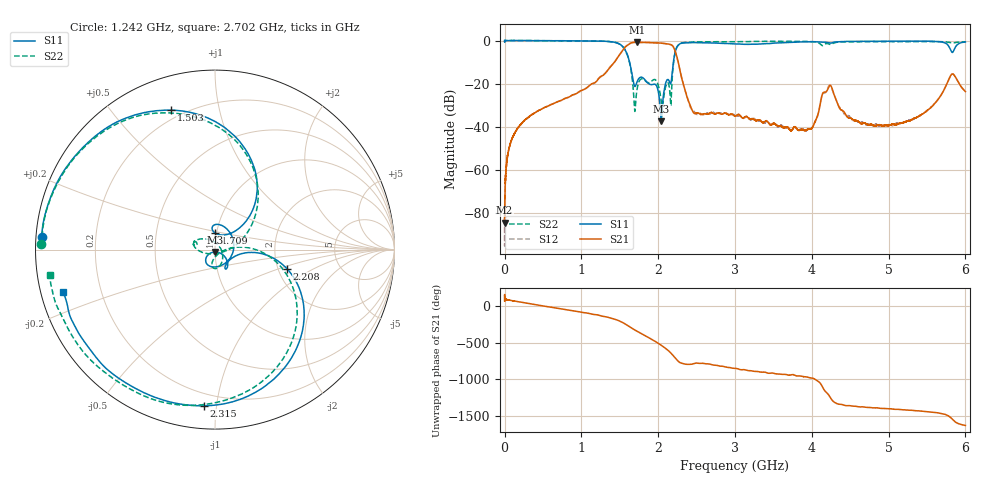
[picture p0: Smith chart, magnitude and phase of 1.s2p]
!Keysight Technologies,N5232A,MY52221221,A.10.65.11
!Date: Sunday, April 23, 2023 11:18:08
!Correction: S11(Full 2 Port(1,4))
!S41(Full 2 Port(1,4))
!S14(Full 2 Port(1,4))
!S44(Full 2 Port(1,4))
!S2P File: Measurements: S11, S41, S14, S44:
# Hz S  RI  R 50
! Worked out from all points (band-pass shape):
!   16001 points, 300 kHz to 6 GHz, reference 50 ohm
!   highest |S21| = -0.83 dB at 1.722 GHz (marker M1); lowest = -84.6 dB at 675 kHz (marker M2)
!   |S21| within 3 dB of the highest: 1.551 GHz to 2.209 GHz (658.2 MHz wide, 35 % of centre)
!   lowest |S11| = -37.5 dB at 2.039 GHz (marker M3), VSWR 1.03, Z = 50 - j1.33 ohm
!   |S11| at or under -10 dB: 1.627 GHz to 2.198 GHz (571.1 MHz wide, 29.9 % of centre)
!   |S22| runs from -32.9 to 0.0 dB; largest |S21 - S12| = 0.024
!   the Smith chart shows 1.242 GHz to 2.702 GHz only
!   S11 on the Smith chart (normalised r, x): 1.242 GHz: 0.02, +0.04; 1.503 GHz: 0.16, +0.72; 1.709 GHz: 0.99, +0.18; 2.208 GHz: 2.23, -0.57; 2.315 GHz: 0.13, -0.93; 2.702 GHz: 0.07, -0.14
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300000  0.999 -0.00352  2.45e-05 6.59e-05  8.74e-05 6.44e-05  0.9988 -0.00308
674981.2  0.9223 0.0318  -5.34e-05 2.5e-05  6.53e-07 -1.69e-05  0.9179 0.042
5.542224e7  0.9858 -0.1449  0.000553 0.00299  0.000502 0.00295  0.986 -0.141
1.780411e8  0.8867 -0.4586  0.00526 0.00818  0.00523 0.00813  0.894 -0.4466
1.000375e9  -0.816 -0.5428  0.00475 -0.0695  0.00649 -0.0679  -0.7934 -0.5667
1.241863e9  -0.9663 0.0703  -0.0925 -0.1079  -0.092 -0.1037  -0.9681 0.0285
1.50285e9  -0.2463 0.7769  -0.4234 0.2386  -0.4193 0.2331  -0.2972 0.762
1.708715e9  0.00118 0.0917  0.8254 0.3764  0.8298 0.3732  -0.0345 -0.0232
1.722214e9  -0.0127 0.106  0.8713 0.257  0.8734 0.251  -0.067 -0.0167
1.877456e9  0.0972 -0.0225  0.2656 -0.8616  0.2678 -0.8536  -0.102 0.0259
2.00045e9  -0.0491 -0.045  -0.75 -0.4556  -0.7498 -0.4571  -0.0697 0.06
2.039448e9  0.000218 -0.0133  -0.8651 -0.0637  -0.8661 -0.0649  0.00324 0.0383
2.139193e9  0.0559 -0.1043  -0.2073 0.7969  -0.2023 0.7989  -0.0157 -0.0925
2.207815e9  0.3997 -0.1053  0.5881 0.2815  0.5917 0.2995  0.3754 -0.1058
2.315059e9  -0.0598 -0.8705  0.0524 -0.1027  0.0482 -0.1071  -0.1997 -0.8653
2.70204e9  -0.845 -0.2343  0.00306 -0.0209  0.00434 -0.0204  -0.9214 -0.144
3.00015e9  -0.8259 0.0693  -0.0118 -0.0132  -0.013 -0.0128  -0.9217 0.1746
4.000225e9  -0.694 0.631  -0.00122 0.00918  -0.00125 0.00932  -0.5475 0.7646
4.237213e9  -0.5492 0.6753  -0.0859 -0.0301  -0.0878 -0.0253  -0.4628 0.6662
5.0003e9  -0.2096 0.9373  0.00826 0.00676  0.00874 0.00688  -0.2002 0.9212
5.826009e9  0.1908 0.4959  -0.0267 -0.1643  -0.0266 -0.1654  0.1785 0.8666
6e9  0.2763 0.8808  -0.0648 0.0093  -0.0652 0.00914  0.2529 0.902
